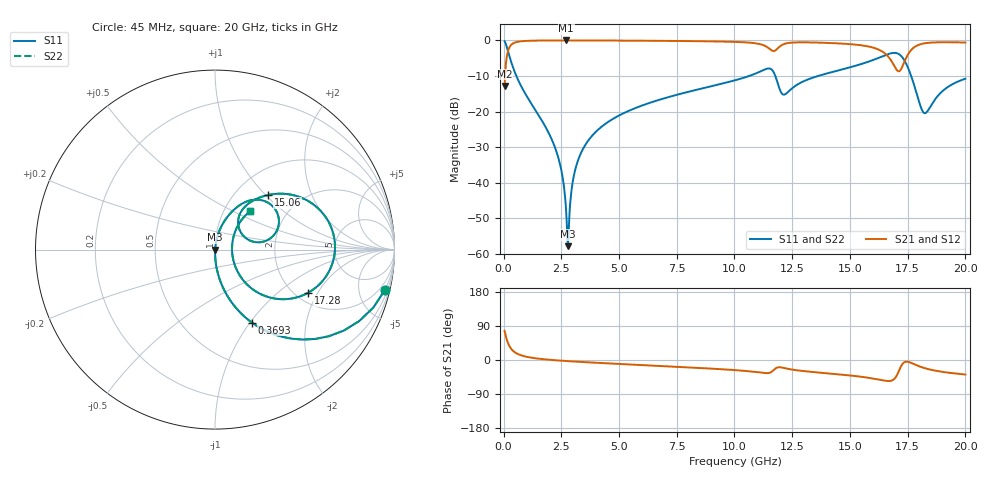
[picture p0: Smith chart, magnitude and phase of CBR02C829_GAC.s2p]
! S-parameter model data by Modelithics Inc.  support@modelithics.com 813-866-6335  Tampa FL USA
! S-Parameter data specifications:
! Substrate: 20-mil Rogers 4350B, substrate thickness, H=0.508mm, Dielectric constant, Er=3.75
! PCB Mounting Pad Footprint: Pad width, PadW=0.32mm , Pad length, PadL=0.37mm , Pad gap, PadG (edge-to-edge)=0.19mm , Reference planes=0.93mm apart
#  GHz  S  MA  R 50
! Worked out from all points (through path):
!   801 points, 45 MHz to 20 GHz, reference 50 ohm
!   highest |S21| = -0.01 dB at 2.714 GHz (marker M1); lowest = -12.8 dB at 45 MHz (marker M2)
!   group delay of S21, straight-line fit = 6.79 ps
!   lowest |S11| = -57.8 dB at 2.789 GHz (marker M3), VSWR 1.00, Z = 50.1 + j0.0158 ohm
!   |S11| at or under -10 dB: 553.7 MHz to 10.64 GHz (10.08 GHz wide, 180 % of centre); 11.77 GHz to 13.62 GHz (1.851 GHz wide, 14.6 % of centre); 17.65 GHz to end of sweep
!   |S22| runs from -57.8 to -0.2 dB; largest |S21 - S12| = 0
!   S11 on the Smith chart (normalised r, x): 45 MHz: 0.99, -8.51; 369.3 MHz: 0.99, -1.02; 15.06 GHz: 1.39, +1.03; 17.28 GHz: 2.32, -1.66; 20 GHz: 1.32, +0.62
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0.045  0.9736 -13.2  0.228 76.8  0.228 76.8  0.9736 -13.2
0.194662  0.7006 -45.7  0.7131 44.3  0.7131 44.3  0.7006 -45.7
0.369269  0.4551 -63.2  0.8898 26.7  0.8898 26.7  0.4551 -63.2
0.8432  0.2027 -79.0  0.9784 10.8  0.9784 10.8  0.2027 -79.0
2.24005  0.03044 -88.5  0.9983 -0.7  0.9983 -0.7  0.03044 -88.5
2.539375  0.01288 -86.5  0.9987 -2.0  0.9987 -2.0  0.01288 -86.5
2.713981  0.003775 -73.4  0.9987 -2.7  0.9987 -2.7  0.003775 -73.4
2.788813  0.001281 7.1  0.9987 -3.0  0.9987 -3.0  0.001281 7.1
3.063194  0.01341 80.4  0.9986 -4.0  0.9986 -4.0  0.01341 80.4
3.387462  0.02764 82.0  0.9982 -5.2  0.9982 -5.2  0.02764 82.0
4.534875  0.07172 79.8  0.9958 -9.0  0.9958 -9.0  0.07172 79.8
6.704981  0.1451 73.7  0.9873 -15.5  0.9873 -15.5  0.1451 73.7
10.0225  0.2751 61.8  0.9537 -26.7  0.9537 -26.7  0.2751 61.8
11.51913  0.4028 31.2  0.7598 -33.7  0.7598 -33.7  0.4028 31.2
12.14272  0.1728 33.1  0.8887 -21.0  0.8887 -21.0  0.1728 33.1
13.36496  0.2974 54.9  0.936 -31.5  0.936 -31.5  0.2974 54.9
15.06114  0.4239 45.9  0.8835 -41.2  0.8835 -41.2  0.4239 45.9
16.68248  0.6463 15.3  0.579 -55.5  0.579 -55.5  0.6463 15.3
17.28113  0.5714 -24.9  0.4367 -10.0  0.4367 -10.0  0.5714 -24.9
17.73012  0.2652 -47.4  0.7768 -9.6  0.7768 -9.6  0.2652 -47.4
18.22899  0.09499 -2.0  0.9095 -21.3  0.9095 -21.3  0.09499 -2.0
20  0.2897 47.5  0.9353 -38.2  0.9353 -38.2  0.2897 47.5
